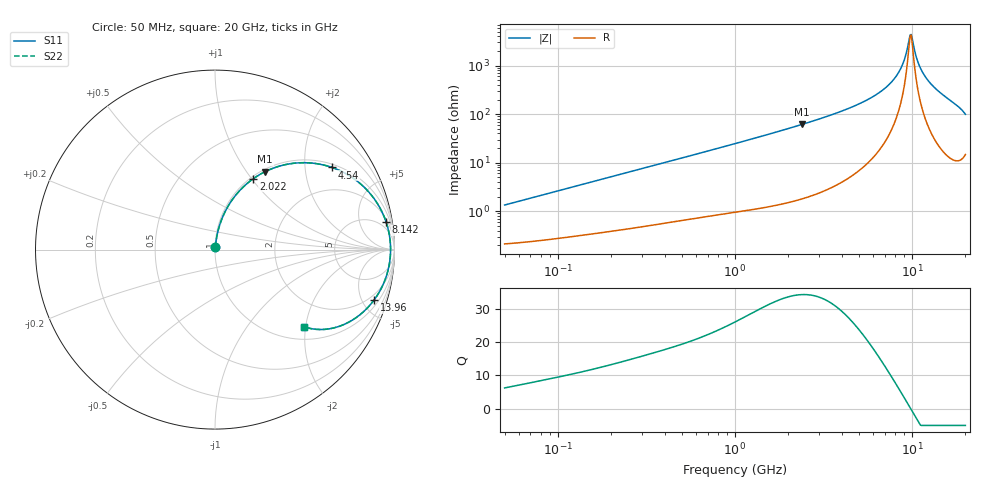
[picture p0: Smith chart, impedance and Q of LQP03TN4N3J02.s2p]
!Murata Part Number: LQP03TN4N3J02
!These Parameters are Measured in Series Mode Connection
!  o--[Z]--o
!Port1  Port2
!  o-------o
!Freq. Start=50[MHz] Stop=20[GHz], 401[Steps]
# Hz S RI R 50
!Freq.(Hz) S11(Real) S11(Imag) S21(Real) S21(Imag) S12(Real) S12(Imag) S22(Real) S22(Imag)
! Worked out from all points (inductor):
!   401 points, 50 MHz to 20 GHz, reference 50 ohm
!   read as one part in series: L = 4.2 nH near 51.52 MHz
!   highest Q = 34.2 at 2.384 GHz (marker M1), where L = 4.09 nH
!   self-resonance near 9.745 GHz
!   S11 on the Smith chart (normalised r, x): 50 MHz: 1.00, +0.03; 2.022 GHz: 1.03, +1.02; 4.54 GHz: 1.11, +2.77; 8.142 GHz: 3, +12; 13.96 GHz: 1.47, -6.11; 20 GHz: 1.30, -1.97
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5e7  0.00229 0.0132  0.9977 -0.0132  0.9977 -0.0132  0.00229 0.0132
1.364002e8  0.00441 0.035  0.9956 -0.035  0.9956 -0.035  0.00441 0.035
3.721004e8  0.0139 0.0916  0.9861 -0.0916  0.9861 -0.0916  0.0139 0.0916
1e9  0.0654 0.2288  0.9346 -0.2288  0.9346 -0.2288  0.0654 0.2288
2.021818e9  0.2144 0.3958  0.7856 -0.3958  0.7856 -0.3958  0.2144 0.3958
2.383959e9  0.2789 0.4341  0.7211 -0.4341  0.7211 -0.4341  0.2789 0.4341
2.728004e9  0.3424 0.46  0.6576 -0.46  0.6576 -0.46  0.3424 0.46
4.539627e9  0.6527 0.4575  0.3473 -0.4575  0.3473 -0.4575  0.6527 0.4575
6.034176e9  0.8295 0.3493  0.1705 -0.3493  0.1705 -0.3493  0.8295 0.3493
7.442007e9  0.9264 0.2182  0.0736 -0.2182  0.0736 -0.2182  0.9264 0.2182
8.141811e9  0.954 0.1517  0.046 -0.1517  0.046 -0.1517  0.954 0.1517
8.774992e9  0.9694 0.0929  0.0306 -0.0929  0.0306 -0.0929  0.9694 0.0929
9.178299e9  0.9751 0.0566  0.0249 -0.0566  0.0249 -0.0566  0.9751 0.0566
9.600142e9  0.9779 0.0197  0.0221 -0.0197  0.0221 -0.0197  0.9779 0.0197
9.892087e9  0.9783 -0.00515  0.0217 0.00515  0.0217 0.00515  0.9783 -0.00515
1.004137e10  0.978 -0.0176  0.022 0.0176  0.022 0.0176  0.978 -0.0176
1.066139e10  0.9735 -0.0674  0.0265 0.0674  0.0265 0.0674  0.9735 -0.0674
1.131968e10  0.9637 -0.117  0.0363 0.117  0.0363 0.117  0.9637 -0.117
1.238412e10  0.9389 -0.1898  0.0611 0.1898  0.0611 0.1898  0.9389 -0.1898
1.396067e10  0.8861 -0.2813  0.1139 0.2813  0.1139 0.2813  0.8861 -0.2813
1.721783e10  0.7278 -0.413  0.2722 0.413  0.2722 0.413  0.7278 -0.413
2e10  0.4978 -0.4305  0.5022 0.4305  0.5022 0.4305  0.4978 -0.4305
